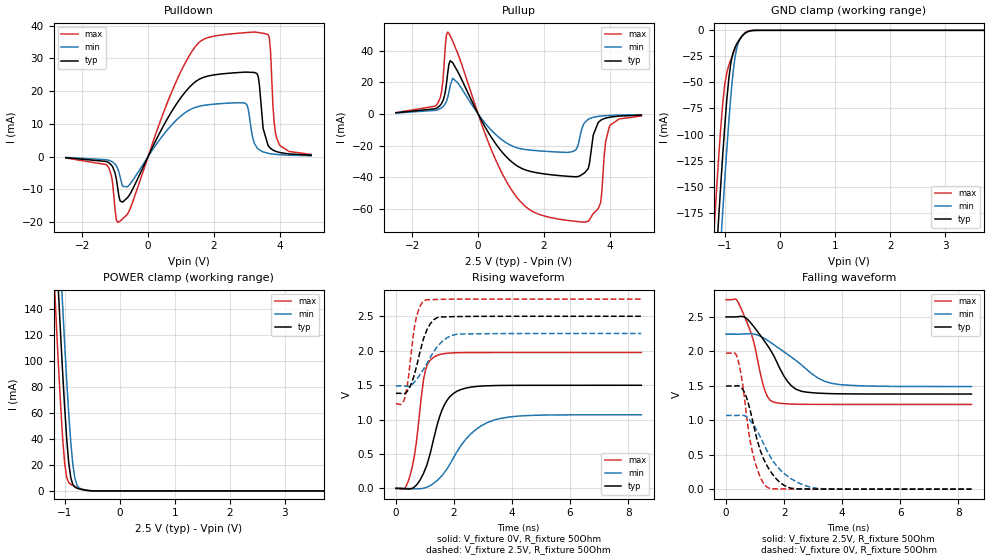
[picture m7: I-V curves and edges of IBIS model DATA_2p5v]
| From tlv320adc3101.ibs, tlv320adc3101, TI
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|   DATA_2p5v
[Model]   DATA_2p5v
Model_type   3-state
Polarity   Non-Inverting
Vmeas = 1.25
Vref = 0
Cref = 5pF
Rref = 1000000
|   typ   min   max
C_comp   1.339pF   1.297pF   1.403pF
[Voltage Range]   2.5   2.25   2.75
[Temperature Range]   27   85   -40
[Pullup Reference]   2.5   2.25   2.75
[Pulldown Reference]   -0   -0   -0
[Power Clamp Reference]   2.5   2.25   2.75
[GND Clamp Reference]   -0   -0   -0
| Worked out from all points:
|   slope of the pulldown table from 0 to 0.375 V, typ, clamps not added: 48.9 ohm
|   slope of the pullup table from 0 to 0.375 V, typ, clamps not added: 27 ohm
|   GND clamp passes 1 mA (typ) near -0.57 V on its own axis
|   POWER clamp passes 1 mA (typ) near -0.68 V on its own axis
|   falling waveform, V_fixture 2.5V, R_fixture 50Ohm: 20-80 % time 950ps typ, 1.42ns min, 569ps max; typ from 2.5 V to 1.38 V
|   rising waveform, V_fixture 0V, R_fixture 50Ohm: 20-80 % time 624ps typ, 1.12ns min, 351ps max; typ from 0 V to 1.5 V
|   rising waveform, V_fixture 2.5V, R_fixture 50Ohm: 20-80 % time 442ps typ, 698ps min, 281ps max; typ from 1.38 V to 2.5 V
|   falling waveform, V_fixture 0V, R_fixture 50Ohm: 20-80 % time 672ps typ, 985ps min, 448ps max; typ from 1.5 V to 0 V
[Pulldown]
|   Voltage   I(typ)   I(min)   I(max)
-2.5V     -290.4uA   -214.8uA   -365.7uA
-1.262V   -1.446mA   -910.1uA   -2.413mA
-887.5mV  -11.91mA   -4.601mA   -19.91mA
-625mV    -12.52mA   -9.186mA   -17.55mA
1.4V      22.56mA    14.92mA    33.12mA
2.975V    25.83mA    16.23mA    37.89mA
3.237V    25.72mA    4.067mA    38.06mA
3.35V     24.5mA     2.362mA    37.92mA
3.688V    2.944mA    981uA      36.32mA
3.837V    1.847mA    772.2uA    10.27mA
3.987V    1.334mA    635.5uA    3.852mA
4.963V    465.5uA    292.7uA    680.2uA
[GND Clamp]
|   Voltage   I(typ)   I(min)   I(max)
-2.5V     -1.51A     -1.565A    -1.451A
-1.188V   -247.1mA   -305mA     -185.9mA
-1.113V   -181.3mA   -238.1mA   -123mA
-1.075V   -149.7mA   -205.6mA   -94.63mA
-1.038V   -119.5mA   -173.7mA   -70.13mA
-1V       -91.25mA   -142.9mA   -51.77mA
-925mV    -45.17mA   -85.97mA   -33.3mA
-887.5mV  -30.41mA   -61.24mA   -27.72mA
-812.5mV  -16.09mA   -25.08mA   -17.97mA
-775mV    -12.25mA   -15.26mA   -13.63mA
-587.5mV  -1.331mA   -1.526mA   -812.9uA
4.963V    0A         0A         0A
[Pullup]
|   Voltage   I(typ)   I(min)   I(max)
-2.5V     743.9uA    600.7uA    889.9uA
-1.225V   4.141mA    2.749mA    6.791mA
-1.113V   6.613mA    3.922mA    14.08mA
-925mV    26.04mA    10.52mA    51.81mA
-775mV    32.47mA    22.59mA    46.13mA
1.1V      -31.59mA   -20.81mA   -50.59mA
2.9V      -39.66mA   -23.55mA   -67.78mA
3.237V    -37.26mA   -5.472mA   -68.46mA
3.725V    -4.034mA   -1.334mA   -56.11mA
3.875V    -2.643mA   -1.069mA   -17.72mA
3.987V    -2.088mA   -928.9uA   -8.26mA
4.963V    -724.7uA   -431.5uA   -1.273mA
[POWER Clamp]
|   Voltage   I(typ)   I(min)   I(max)
-2.5V     1.483A     1.534A     1.43A
-1.188V   220.4mA    274.7mA    162.5mA
-1.15V    187.2mA    241.2mA    129.8mA
-1.113V   154.7mA    208.3mA    98.28mA
-1.075V   123.3mA    176.1mA    68.74mA
-1.038V   93.33mA    144.8mA    42.52mA
-1V       65.52mA    114.6mA    22.2mA
-925mV    22.05mA    60.2mA     6.551mA
-850mV    4.938mA    20.68mA    4.11mA
-775mV    2.1mA      4.545mA    2.722mA
-437.5mV  17.61uA    34.89uA    9.8uA
4.963V    0A         0A         0A
[Ramp]
R_load = 50
|   typ   min   max
dV/dt_r   0.898625/6.2424e-010   0.641668/1.11989e-009   1.1843/3.51155e-010
dV/dt_f   0.671697/9.49615e-010  0.456543/1.4248e-009   0.9125/5.69143e-010
[Falling Waveform]
V_fixture = 2.5V
V_fixture_min = 2.25V
V_fixture_max = 2.75V
R_fixture = 50Ohm
C_fixture = 0F
|   Time   V(typ)   V(min)   V(max)
0s        2.5V       2.25V      2.75V
470.4ps   2.506V     2.25V      2.667V
891.1ps   2.393V     2.255V     2.228V
1.345ns   2.135V     2.181V     1.423V
1.618ns   1.955V     2.106V     1.266V
2.114ns   1.566V     1.958V     1.238V
2.612ns   1.419V     1.799V     1.232V
3.16ns    1.394V     1.614V     1.23V
3.929ns   1.384V     1.517V     1.23V
8.458ns   1.381V     1.489V     1.229V
[Rising Waveform]
V_fixture = 0V
V_fixture_min = 0V
V_fixture_max = 0V
R_fixture = 50Ohm
C_fixture = 0F
|   Time   V(typ)   V(min)   V(max)
0s        12.33uV    -14.73uV   363.1uV
470.4ps   -8.015mV   -3.267mV   163.5mV
641.4ps   22.31mV    -6.152mV   483.9mV
1.016ns   285.8mV    10.02mV    1.715V
1.345ns   794.4mV    88.91mV    1.916V
1.666ns   1.21V      228mV      1.958V
1.983ns   1.379V     442.2mV    1.969V
2.563ns   1.469V     784.2mV    1.973V
3.398ns   1.493V     994.6mV    1.974V
8.458ns   1.498V     1.069V     1.974V
[Rising Waveform]
V_fixture = 2.5V
V_fixture_min = 2.25V
V_fixture_max = 2.75V
R_fixture = 50Ohm
C_fixture = 0F
|   Time   V(typ)   V(min)   V(max)
0s        1.381V     1.489V     1.23V
186.7ps   1.378V     1.489V     1.224V
308.6ps   1.378V     1.486V     1.319V
400ps     1.416V     1.482V     1.519V
512.8ps   1.503V     1.496V     1.914V
703.9ps   1.763V     1.579V     2.484V
1.016ns   2.247V     1.777V     2.736V
1.417ns   2.48V      2.054V     2.745V
2.077ns   2.495V     2.237V     2.749V
8.458ns   2.5V       2.25V      2.75V
[Falling Waveform]
|Gnd
V_fixture = 0V
V_fixture_min = 0V
V_fixture_max = 0V
R_fixture = 50Ohm
C_fixture = 0F
|   Time   V(typ)   V(min)   V(max)
0s        1.498V     1.069V     1.974V
400ps     1.501V     1.07V      1.89V
516.6ps   1.476V     1.073V     1.67V
638.3ps   1.401V     1.066V     1.308V
891.1ps   1.036V     964.5mV    573.8mV
1.141ns   616.9mV    791.1mV    214.2mV
1.425ns   330.4mV    545.2mV    25.72mV
1.983ns   59.53mV    235.9mV    3.218mV
2.923ns   2.343mV    28.18mV    698.8uV
8.458ns   -3.293uV   18.05uV    -3.466uV
